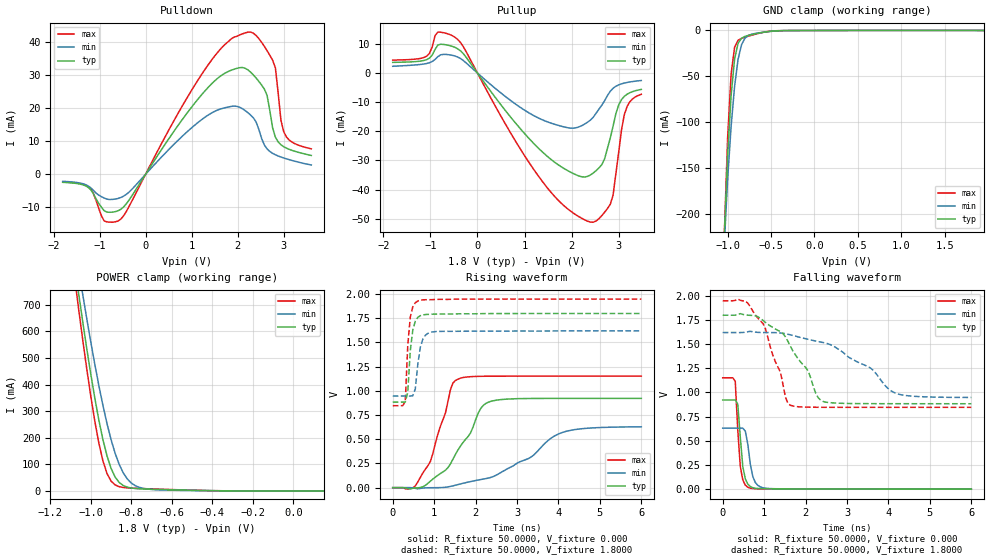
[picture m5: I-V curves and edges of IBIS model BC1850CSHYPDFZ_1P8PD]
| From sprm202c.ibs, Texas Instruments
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|   Model BC1850CSHYPDFZ_1P8PD
[Model]   BC1850CSHYPDFZ_1P8PD
Model_type   I/O
Polarity   Non-Inverting
Enable   Active-Low
Vinl =   0.8500V
Vinh =   0.9800V
Vmeas =   0.9000V
Cref =  15.0000pF
Rref = 100.0000M
Vref =  0.000V
C_comp   1.3000pF   1.4700pF   1.1000pF
[Model Spec]
|   typ   min   max
Vinh   0.98V   0.86V   1.1V
Vinl   0.85V   0.70V   0.91V
[Temperature Range]   25.0000   0.1250k   -40.0000
[Voltage Range]   1.8000V   1.6200V   1.9500V
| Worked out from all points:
|   slope of the pulldown table from 0 to 0.27 V, typ, clamps not added: 46 ohm
|   slope of the pullup table from 0 to 0.27 V, typ, clamps not added: 44.9 ohm
|   GND clamp passes 1 mA (typ) near -0.52 V on its own axis
|   POWER clamp passes 1 mA (typ) near -0.39 V on its own axis
|   rising waveform, R_fixture 50.0000, V_fixture 0.000: 20-80 % time 751ps typ, 1.31ns min, 493ps max; typ from 0 V to 0.922 V
|   rising waveform, R_fixture 50.0000, V_fixture 1.8000: 20-80 % time 106ps typ, 132ps min, 96ps max; typ from 0.883 V to 1.8 V
|   falling waveform, R_fixture 50.0000, V_fixture 0.000: 20-80 % time 119ps typ, 142ps min, 101ps max; typ from 0.922 V to 0 V
|   falling waveform, R_fixture 50.0000, V_fixture 1.8000: 20-80 % time 751ps typ, 1.26ns min, 522ps max; typ from 1.8 V to 0.883 V
[Pulldown]
| voltage   I(typ)   I(min)   I(max)
-1.8V     -2.432mA   -2.13mA    -2.324mA
-1.2V     -4.535mA   -3.994mA   -4.328mA
-900mV    -11.04mA   -7.186mA   -14.12mA
-540mV    -10.64mA   -7.052mA   -13.61mA
1.32V     25.76mA    17.6mA     32.41mA
2.22V     31.69mA    18.71mA    43.1mA
2.58V     25.85mA    8.892mA    38.8mA
2.76V     14.04mA    6.343mA    34.57mA
2.82V     11.26mA    5.911mA    32.25mA
2.94V     8.959mA    5.237mA    16.42mA
3.06V     7.924mA    4.688mA    11.3mA
3.6V      5.706mA    2.822mA    7.711mA
[Pullup]
| voltage   I(typ)   I(min)   I(max)
-1.8V     3.669mA    2.32mA     4.446mA
-1.08V    4.598mA    3.276mA    5.78mA
-840mV    9.631mA    5.639mA    14.06mA
-420mV    8.322mA    5.5mA      11.54mA
1.32V     -26.18mA   -15.62mA   -35.92mA
1.98V     -34.04mA   -18.91mA   -47.41mA
2.4V      -34.97mA   -16.12mA   -51.17mA
2.64V     -31.45mA   -11.07mA   -48.94mA
2.82V     -22.35mA   -6.261mA   -45.06mA
2.88V     -18.23mA   -5.221mA   -41.92mA
3.12V     -7.968mA   -3.432mA   -14.2mA
3.48V     -5.617mA   -2.562mA   -7.289mA
[GND_clamp]
| voltage   I(typ)   I(min)   I(max)
-1.8V     -5.333A    -4.658A    -5.852A
-1.04V    -227mA     -235.1mA   -226.5mA
-1V       -135.9mA   -161.8mA   -116.4mA
-960mV    -70.64mA   -104.3mA   -47.39mA
-920mV    -31.06mA   -60.7mA    -18.2mA
-880mV    -13.96mA   -31.42mA   -10.74mA
-840mV    -8.411mA   -15.42mA   -8.563mA
-800mV    -6.408mA   -8.312mA   -7.264mA
-760mV    -5.281mA   -5.37mA    -6.127mA
-560mV    -1.528mA   -1.553mA   -1.454mA
-440mV    -390.7uA   -531uA     -281uA
1.95V     0A         0A         0A
[POWER_clamp]
| voltage   I(typ)   I(min)   I(max)
-1.8V     5.299A     4.889A     5.644A
-1.08V    850.3mA    929.8mA    802.1mA
-1.06V    742mA      833.5mA    683.7mA
-1.04V    636.9mA    739.4mA    569mA
-1V       438.9mA    559.8mA    355.9mA
-960mV    265.5mA    395.4mA    179mA
-940mV    192.6mA    321mA      112.6mA
-920mV    131.8mA    253.2mA    65.44mA
-880mV    52.35mA    141.8mA    22.62mA
-820mV    14.23mA    45.21mA    11.42mA
-740mV    7.291mA    9.432mA    8.657mA
150mV     0A         0A         0A
[Ramp]
| variable   typ   min   max
dV/dt_r   0.5530/0.7482n   0.3780/1.3691n   0.6904/0.4974n
dV/dt_f   0.5489/0.7495n   0.4038/1.3083n   0.6605/0.5247n
R_load = 50.0000
[Rising Waveform]
R_fixture = 50.0000
V_fixture = 0.000
V_fixture_min = 0.000
V_fixture_max = 0.000
| time   V(typ)   V(min)   V(max)
0s        2.482uV    1.452uV    3.766uV
484.8ps   -6.728mV   -2.211mV   -1.863mV
848.5ps   43.93mV    -1.387mV   225.5mV
1.273ns   179.8mV    4.059mV    770.4mV
1.394ns   245.5mV    12.64mV    1.012V
1.576ns   388.8mV    31.56mV    1.119V
2.121ns   815.1mV    83.47mV    1.149V
2.364ns   890.2mV    105mV      1.15V
4.121ns   921.2mV    573.2mV    1.151V
6ns       921.6mV    627.7mV    1.151V
[Rising Waveform]
R_fixture = 50.0000
V_fixture = 1.8000
V_fixture_min = 1.6200
V_fixture_max = 1.9500
| time   V(typ)   V(min)   V(max)
0s        882.6mV    945.5mV    845.6mV
303ps     881.8mV    946mV      890.1mV
363.6ps   985.8mV    945.6mV    1.469V
424.2ps   1.412V     945.2mV    1.759V
484.8ps   1.627V     948.7mV    1.867V
545.5ps   1.718V     1.02V      1.908V
606.1ps   1.757V     1.274V     1.927V
727.3ps   1.782V     1.532V     1.938V
969.7ps   1.79V      1.608V     1.94V
6ns       1.798V     1.618V     1.946V
[Falling Waveform]
R_fixture = 50.0000
V_fixture = 0.000
V_fixture_min = 0.000
V_fixture_max = 0.000
| time   V(typ)   V(min)   V(max)
0s        921.7mV    630.3mV    1.151V
303ps     922.2mV    630.3mV    1.114V
363.6ps   877.9mV    630.3mV    610mV
424.2ps   538.6mV    630.6mV    236.3mV
484.8ps   233.1mV    630.4mV    95.73mV
545.5ps   106.4mV    599.4mV    41.75mV
606.1ps   51.6mV     463.8mV    19.91mV
727.3ps   14.84mV    128.8mV    6.115mV
969.7ps   5.327mV    15.01mV    3.802mV
6ns       53.06uV    376.9uV    3.813uV
[Falling Waveform]
R_fixture = 50.0000
V_fixture = 1.8000
V_fixture_min = 1.6200
V_fixture_max = 1.9500
| time   V(typ)   V(min)   V(max)
0s        1.798V     1.619V     1.946V
545.5ps   1.8V       1.621V     1.942V
969.7ps   1.745V     1.619V     1.713V
1.394ns   1.627V     1.614V     1.207V
1.515ns   1.573V     1.607V     950.2mV
1.636ns   1.474V     1.595V     866mV
2.424ns   905.9mV    1.515V     846mV
3.576ns   883.6mV    1.249V     845.7mV
4.182ns   883.1mV    990.4mV    845.6mV
6ns       882.7mV    947.4mV    845.6mV
